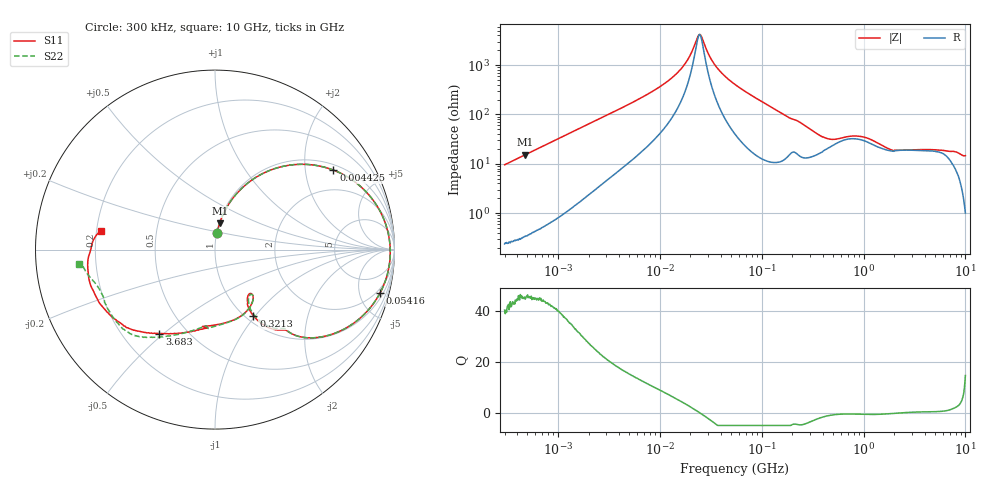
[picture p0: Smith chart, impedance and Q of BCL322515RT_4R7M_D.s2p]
! S-Parameter Data Generated by TDK Corporation
! Copyright(C) 2024 TDK Corporation.
! All Rights Reserved.
! TDK P/N: BCL322515RT-4R7M-D (SMD / SMT Inductor (Coil))
! Property: L=4.7uH at 1MHz
! Size(LxWxT): 3.2x2.5x1.5mm
! Model Type: s2p (Touchstone File Format Version 1.0)
! Frequency: DC=Yes Start=0.3MHz Stop=10000MHz 802points Log-sweep
! Model Generated on May 28, 2024
! Terms and conditions regarding TDK Simulation Models:
! 1)This simulation model is being provided solely for informational
!  purposes. Please refer to the specifications of the products in
!  terms of detailed characteristics of such products.
! 2)In no event shall TDK Corporation of any of its subsidiaries be
!  liable for any loss or damage arising, directly or indirectly,
!  from any information contained in this simulation model, including,
!  but not limited to loss or damages arising from any inaccuracies,
!  omissions or errors in connection with such information.
! 3)Any and all copyrights on this simulation model are owned by
!  TDK Corporation.  Duplication or redistribution of this simulation
!  model without prior written permission from TDK Corporation
!  is prohibited.
! 4)This simulation model is subject to any modification or change
!  without any prior notice.
! 5)Neither TDK Corporation nor any of its subsidiaries shall make any
!  warranty, express or implied, including but not limited to the
!  correctness, implied warranties of merchantability and fitness for
!  a particular purpose with respect to this simulation models.
! 6)The use of this simulation model shall be deemed to have consented
!  to the terms and conditions hereof.
! Port Assignments:
!  1 ---@@@--- 2
! Applicable Conditions:
!  Temperature = 25 degC
!  DC Bias Current = 0 A
!  Small Signal Operation
# Hz S MA R 50
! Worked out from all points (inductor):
!   801 points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, 300 kHz to 10 GHz, reference 50 ohm
!   read as one part in series: L = 5.06 uH near 318.3 kHz
!   highest Q = 45.5 at 478.9 kHz (marker M1), where L = 5.07 uH
!   self-resonance near 24.61 MHz
!   S11 on the Smith chart (normalised r, x): 300 kHz: 1.01, +0.19; 4.425 MHz: 1.18, +2.84; 54.16 MHz: 1.47, -7.42; 321.3 MHz: 1.09, -0.98; 3.683 GHz: 0.35, -0.48; 10 GHz: 0.22, +0.08
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300000  0.09266 82.9  0.9933 -5.6  0.9932 -5.5  0.0929 83.0
478871  0.1488 79.9  0.9852 -8.7  0.9856 -8.7  0.1489 80.0
1713600  0.4716 59.9  0.866 -28.2  0.8663 -28.2  0.4716 59.9
4425256  0.7949 33.9  0.5602 -52.6  0.5603 -52.6  0.795 33.9
9671944  0.9342 15.2  0.2692 -68.5  0.2693 -68.5  0.9344 15.2
1.672204e7  0.9693 5.5  0.1065 -70.8  0.1066 -70.8  0.9694 5.4
2.473055e7  0.9766 -0.8  0.02338 2.5  0.02338 2.5  0.9767 -0.8
3.511624e7  0.9729 -6.5  0.09918 70.4  0.09924 70.5  0.9731 -6.6
5.416364e7  0.9506 -14.8  0.2301 69.5  0.2301 69.5  0.9506 -14.8
5.477226e7  0.9496 -15.0  0.2338 69.3  0.2339 69.4  0.9497 -15.0
8.740098e7  0.8864 -26.4  0.4063 59.7  0.4064 59.7  0.8862 -26.4
1.389026e8  0.7543 -40.4  0.5968 44.7  0.597 44.7  0.7533 -40.5
3.126428e8  0.4372 -59.6  0.7943 16.1  0.7946 16.1  0.4387 -58.8
3.212744e8  0.426 -59.9  0.7971 15.1  0.7974 15.1  0.4277 -59.1
5.82867e8  0.3168 -50.6  0.7546 -2.5  0.7549 -2.5  0.3232 -50.7
9.445544e8  0.381 -61.1  0.7183 -8.1  0.7185 -8.2  0.3822 -61.2
1.767019e9  0.4237 -92.7  0.7482 -23.4  0.7484 -23.5  0.4266 -90.0
3.682634e9  0.5615 -123.5  0.6267 -54.1  0.627 -54.2  0.566 -120.7
5.099159e9  0.6472 -137.0  0.5338 -67.9  0.5339 -68.0  0.6594 -133.7
6.576072e9  0.6877 -147.6  0.4951 -79.9  0.495 -80.1  0.6817 -146.5
8.322921e9  0.7175 -170.2  0.4331 -100.0  0.4338 -100.2  0.699 -165.4
1e10  0.6451 170.8  0.3445 -111.5  0.3443 -111.7  0.7645 -173.8
